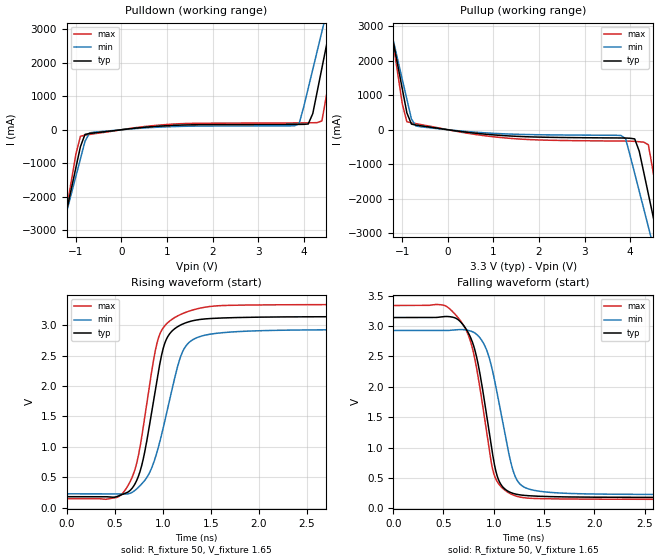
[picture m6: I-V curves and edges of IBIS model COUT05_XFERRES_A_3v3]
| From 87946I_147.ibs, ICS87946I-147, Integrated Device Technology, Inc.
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[Model] COUT05_XFERRES_A_3v3
Model_type   Output
Polarity   Non-Inverting
|   typ   min   max
C_comp   2pF   1.5pF   2.5pF
Vmeas = 1.75V
Rref = 50
Vref = 1.65V
|   typ   min   max
[Voltage range]   3.3V   3.135V   3.465V
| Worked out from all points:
|   slope of the pulldown table from 0 to 0.495 V, typ, clamps not added: 6.88 ohm
|   slope of the pullup table from 0 to 0.495 V, typ, clamps not added: 5.83 ohm
|   rising waveform, R_fixture 50, V_fixture 1.65: 20-80 % time 201ps typ, 255ps min, 203ps max; typ from 0.181 V to 3.14 V
|   falling waveform, R_fixture 50, V_fixture 1.65: 20-80 % time 180ps typ, 198ps min, 195ps max; typ from 3.14 V to 0.181 V
[pulldown]
|Voltage   I (typ)   I (min)   I (max)
-3.3V     -15.53A    -13.39A    -19.08A
-1.3V     -3.015A    -2.955A    -3.131A
-1V       -1.131A    -1.388A    -725.6mA
-800mV    -139.2mA   -344.2mA   -162.8mA
200mV     32.31mA    23.73mA    41.9mA
3.9V      159.3mA    180.5mA    204.1mA
4.2V      482.4mA    1.8A       208mA
4.4V      1.836A     2.927A     263.7mA
4.6V      3.193A     4.056A     1.89A
4.7V      3.873A     4.622A     2.759A
4.8V      4.554A     5.188A     3.63A
6.6V      17.06A     15.56A     19.6A
[pullup]
|Voltage   I (typ)   I (min)   I (max)
-3.3V     16.98A     14.61A     20.9A
-1.3V     3.243A     3.171A     3.379A
-1V       1.177A     1.453A     739.5mA
-800mV    162.5mA    308.2mA    200.5mA
3.8V      -238.9mA   -166.8mA   -327.9mA
3.9V      -241.3mA   -257.1mA   -328.9mA
4.1V      -265.6mA   -1.266A    -337.6mA
4.4V      -1.864A    -2.816A    -435.8mA
4.6V      -3.109A    -3.852A    -1.975A
4.7V      -3.731A    -4.37A     -2.771A
4.8V      -4.354A    -4.888A    -3.566A
6.6V      -15.57A    -14.23A    -17.87A
[Ramp]
|   typ   min   max
dV/dt_r   2.374/0.330n   2.163/0.407n   2.561/0.368n
dV/dt_f   2.381/0.289n   2.171/0.307n   2.565/0.334n
[Rising Waveform]
R_fixture = 50
V_fixture = 1.65
V_fixture_max = 1.73
V_fixture_min = 1.57
C_fixture = 0.0p
| Time   typ   min   max
0s        180.7mV    228.1mV    148.5mV
524.8ps   184.1mV    227.8mV    170.1mV
697ps     355.4mV    267.5mV    563.7mV
799.5ps   819.2mV    423.5mV    1.35V
947.1ps   2.168V     952.1mV    2.747V
1.033ns   2.751V     1.504V     3.011V
1.16ns    2.979V     2.351V     3.156V
1.279ns   3.059V     2.722V     3.233V
1.542ns   3.112V     2.862V     3.315V
3.997ns   3.14V      2.927V     3.339V
[Falling Waveform]
R_fixture = 50
V_fixture = 1.65
V_fixture_max = 1.73
V_fixture_min = 1.57
C_fixture = 0.0p
| Time   typ   min   max
0s        3.141V     2.927V     3.339V
508.4ps   3.157V     2.927V     3.341V
717.5ps   2.969V     2.938V     2.958V
836.4ps   2.438V     2.854V     2.242V
996.3ps   814.4mV    2.2V       594.2mV
1.062ns   419.3mV    1.65V      376.2mV
1.177ns   254.8mV    710.3mV    231.3mV
1.275ns   218.5mV    378.8mV    180.8mV
1.513ns   195.2mV    270mV      158.2mV
3.997ns   180.7mV    228.1mV    148.5mV
